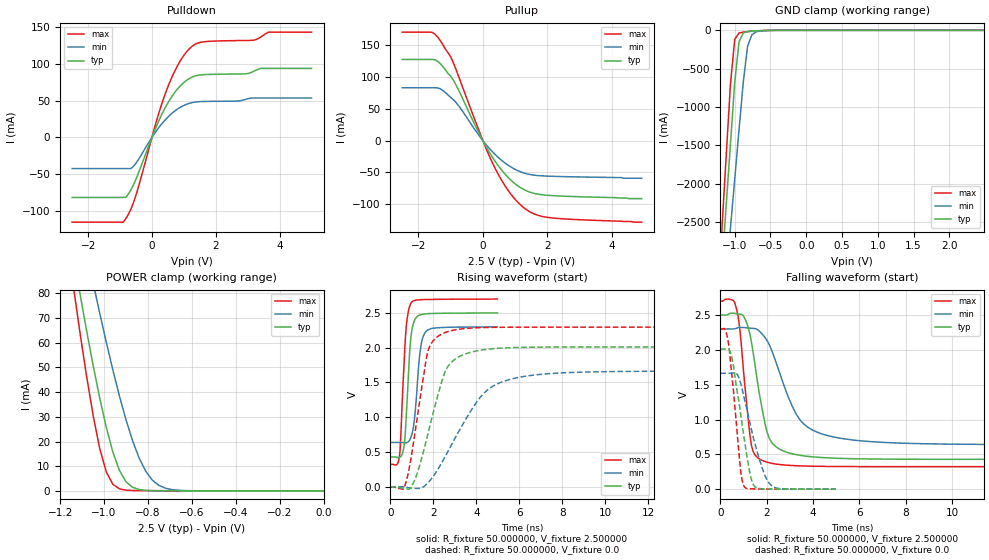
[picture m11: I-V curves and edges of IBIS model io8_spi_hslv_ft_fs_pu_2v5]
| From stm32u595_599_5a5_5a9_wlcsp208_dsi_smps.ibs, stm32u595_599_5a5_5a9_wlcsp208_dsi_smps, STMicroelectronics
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|   Model io8_spi_hslv_ft_fs_pu_2v5
[Model]  io8_spi_hslv_ft_fs_pu_2v5
Model_type I/O
Polarity   Non-Inverting
Enable   Active-Low
Vinl =   0.750000V
Vinh =   1.750000V
Vmeas =  1.250000V
Cref =   50.000000pF
Rref =   100.000000M
Vref =   0.0V
C_comp   3.438200pF   3.436700pF   3.473300pF
[Temperature Range]   25.000000   0.140000k   -40.000000
[Pullup Reference]   2.500000V   2.300000V   2.700000V
[Pulldown Reference]   0.0V   0.0V   0.0V
[POWER Clamp Reference]   2.500000V   2.300000V   2.700000V
[GND Clamp Reference]   0.0V   0.0V   0.0V
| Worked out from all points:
|   slope of the pulldown table from 0 to 0.375 V, typ, clamps not added: 10.1 ohm
|   slope of the pullup table from 0 to 0.375 V, typ, clamps not added: 11.7 ohm
|   GND clamp passes 1 mA (typ) near -0.50 V on its own axis
|   POWER clamp passes 1 mA (typ) near -0.85 V on its own axis
|   rising waveform, R_fixture 50.000000, V_fixture 2.500000: 20-80 % time 228ps typ, 275ps min, 224ps max; typ from 0.428 V to 2.5 V
|   rising waveform, R_fixture 50.000000, V_fixture 0.0: 20-80 % time 1.04ns typ, 1.94ns min, 684ps max; typ from 0 V to 2.01 V
|   falling waveform, R_fixture 50.000000, V_fixture 2.500000: 20-80 % time 645ps typ, 1.26ns min, 407ps max; typ from 2.5 V to 0.428 V
|   falling waveform, R_fixture 50.000000, V_fixture 0.0: 20-80 % time 550ps typ, 767ps min, 384ps max; typ from 2.01 V to 0 V
[Pulldown]
|Voltage   I(typ)   I(min)   I(max)
-2.5V     -81.61mA   -42.31mA   -115.3mA
-900mV    -81.61mA   -42.31mA   -115.3mA
-820mV    -81.42mA   -42.31mA   -110.6mA
-500mV    -56.95mA   -35.08mA   -78.57mA
140mV     15.18mA    9.02mA     22.02mA
460mV     44mA       25.98mA    64.37mA
860mV     68.91mA    40.27mA    102.2mA
1.26V     82.21mA    47.42mA    124mA
1.66V     85.53mA    48.99mA    130.3mA
3.18V     89.84mA    53.63mA    132.3mA
3.66V     94mA       53.63mA    143.4mA
5V        94mA       53.63mA    143.4mA
[Pullup]
|Voltage   I(typ)   I(min)   I(max)
-2.5V     127.4mA    82.99mA    170.4mA
-1.56V    127.4mA    82.99mA    169.7mA
-1.32V    120.7mA    81.18mA    156.8mA
-1V       101.3mA    67.87mA    131.8mA
-920mV    95.41mA    64.46mA    122.6mA
-40mV     3.893mA    2.628mA    5.181mA
360mV     -30.97mA   -20.78mA   -41.56mA
760mV     -56.64mA   -37.85mA   -76.55mA
1.24V     -75.99mA   -50.28mA   -104.1mA
1.64V     -83.42mA   -54.54mA   -116.1mA
2.04V     -85.88mA   -55.77mA   -120.6mA
4.92V     -91mA      -59mA      -128mA
[GND_clamp]
|Voltage   I(typ)   I(min)   I(max)
-2.5V     -9.641A    -9.693A    -9.352A
-1.18V    -3.114A    -3.874A    -2.614A
-1.12V    -2.301A    -3.23A     -1.656A
-1.06V    -1.489A    -2.587A    -706.2mA
-1V       -685.8mA   -1.945A    -119.3mA
-940mV    -149.7mA   -1.304A    -34.73mA
-880mV    -35.54mA   -672.6mA   -23.06mA
-820mV    -16.19mA   -206.4mA   -17.27mA
-760mV    -10.58mA   -57.55mA   -12.41mA
-700mV    -7.152mA   -18.74mA   -8.24mA
-400mV    -103.3uA   -378.5uA   -41.74uA
2.48V     0A         13.22nA    0A
[POWER_clamp]
|Voltage   I(typ)   I(min)   I(max)
-2.49V    881.1mA    773.1mA    1.07A
-1.14V    95.32mA    122.8mA    82.93mA
-1.11V    79.97mA    109.7mA    64.26mA
-1.05V    50.95mA    84.3mA     30.69mA
-1.02V    37.7mA     72.08mA    17.29mA
-990mV    25.79mA    60.29mA    7.738mA
-930mV    8.312mA    38.47mA    853.1uA
-900mV    3.712mA    28.81mA    313.6uA
-840mV    566.2uA    13.29mA    123.7uA
-780mV    119.1uA    4.365mA    94.04uA
-660mV    38.99uA    251.5uA    57.77uA
0V        0A         18.93nA    0A
[Ramp]
| variable   typ   min   max
dV/dt_r  1.20644/1.04128n   0.99765/1.94097n   1.37763/0.68348n
dV/dt_f  1.24312/0.64384n   0.99705/1.25306n   1.42607/0.40578n
R_load = 50.000000
[Rising Waveform]
R_fixture= 50.000000
V_fixture= 2.500000
V_fixture_min= 2.300000
V_fixture_max= 2.700000
|time   V(typ)   V(min)   V(max)
0s        428.1mV    638.2mV    323.3mV
420.4ps   421.7mV    638.2mV    426mV
470.5ps   429.7mV    638.2mV    608.8mV
640.6ps   583.7mV    634.4mV    1.758V
770.8ps   1.171V     635.4mV    2.381V
971ps     2.176V     722.2mV    2.645V
1.121ns   2.389V     964mV      2.679V
1.401ns   2.474V     1.976V     2.69V
1.622ns   2.486V     2.218V     2.692V
4.985ns   2.5V       2.3V       2.7V
[Rising Waveform]
R_fixture= 50.000000
V_fixture= 0.0
V_fixture_min= 0.0
V_fixture_max= 0.0
|time   V(typ)   V(min)   V(max)
0s        439.3uV    552uV      505.8uV
640.6ps   -23.62mV   -549.3uV   -14.87mV
840.8ps   -33.21mV   -13.14mV   205.5mV
1.081ns   58.38mV    -21.05mV   637.8mV
1.762ns   776.9mV    61.39mV    1.961V
2.563ns   1.663V     441.1mV    2.219V
3.163ns   1.865V     783.7mV    2.264V
4.244ns   1.966V     1.308V     2.289V
5.886ns   2.003V     1.568V     2.295V
19.94ns   2.011V     1.663V     2.296V
[Falling Waveform]
R_fixture= 50.000000
V_fixture= 2.500000
V_fixture_min= 2.300000
V_fixture_max= 2.700000
|time   V(typ)   V(min)   V(max)
0s        2.5V       2.3V       2.7V
680.7ps   2.52V      2.308V     2.606V
840.8ps   2.512V     2.322V     2.293V
1.121ns   2.399V     2.317V     1.267V
1.401ns   1.988V     2.309V     554.5mV
1.922ns   951mV      2.179V     398.2mV
2.322ns   631.5mV    1.897V     365.5mV
3.403ns   488.1mV    1.01V      335.2mV
4.685ns   448.8mV    764.9mV    326.7mV
19.94ns   428.1mV    638.2mV    323.3mV
[Falling Waveform]
R_fixture= 50.000000
V_fixture= 0.0
V_fixture_min= 0.0
V_fixture_max= 0.0
|time   V(typ)   V(min)   V(max)
0s        2.011V     1.663V     2.296V
190.2ps   2.011V     1.663V     2.294V
340.3ps   2.017V     1.663V     2.112V
530.5ps   1.834V     1.666V     1.524V
870.9ps   1.092V     1.525V     282.1mV
1.041ns   700.2mV    1.287V     32.16mV
1.431ns   61.63mV    729.6mV    4.507mV
1.892ns   5.386mV    223.4mV    2.517mV
2.182ns   3.414mV    59.01mV    2.05mV
4.985ns   439.3uV    552uV      505.8uV
